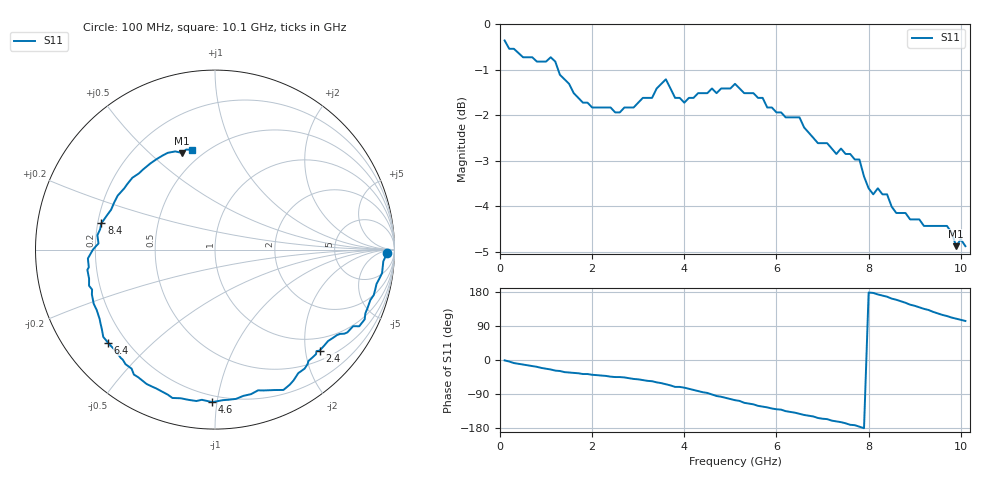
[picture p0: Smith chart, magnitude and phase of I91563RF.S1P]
!	IAM-91563 RF Port S PARAMETERS
!	Vd = 3 V LAST UPDATED 3-12-96
# ghz	s ma r	50
! Freq	RF(Mag)	RF(Ang)
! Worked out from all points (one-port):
!   101 points, 100 MHz to 10.1 GHz, reference 50 ohm
!   lowest |S11| = -4.9 dB at 9.9 GHz (marker M1), VSWR 3.65, Z = 19.9 + j31.8 ohm
!   |S11| at or under -10 dB: nowhere
!   S11 on the Smith chart (normalised r, x): 100 MHz: 41, -18; 2.4 GHz: 0.70, -2.29; 4.6 GHz: 0.16, -0.97; 6.4 GHz: 0.13, -0.37; 8.4 GHz: 0.21, +0.11; 10.1 GHz: 0.43, +0.70
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0.1  0.96 -1.0
0.3  0.94 -8.0
1.1  0.92 -25.0
1.4  0.87 -32.0
1.8  0.82 -37.0
2.4  0.81 -44.0
2.6  0.8 -45.0
3.3  0.83 -56.0
3.6  0.87 -64.0
3.8  0.83 -71.0
3.9  0.83 -71.0
4.6  0.85 -91.0
5.1  0.86 -106.0
5.6  0.83 -121.0
6.4  0.79 -139.0
6.9  0.74 -153.0
7.1  0.74 -156.0
7.4  0.73 -164.0
7.6  0.72 -171.0
7.7  0.71 -172.0
7.9  0.68 -180.0
8.1  0.65 177.0
8.4  0.65 167.0
8.9  0.61 146.0
9.3  0.6 132.0
9.6  0.6 119.0
9.9  0.57 109.0
10.1  0.57 103.0
